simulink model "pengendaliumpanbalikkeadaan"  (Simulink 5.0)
settings: Solver=ode45  StartTime=0.0  StopTime=8.0  RelTol=1e-3

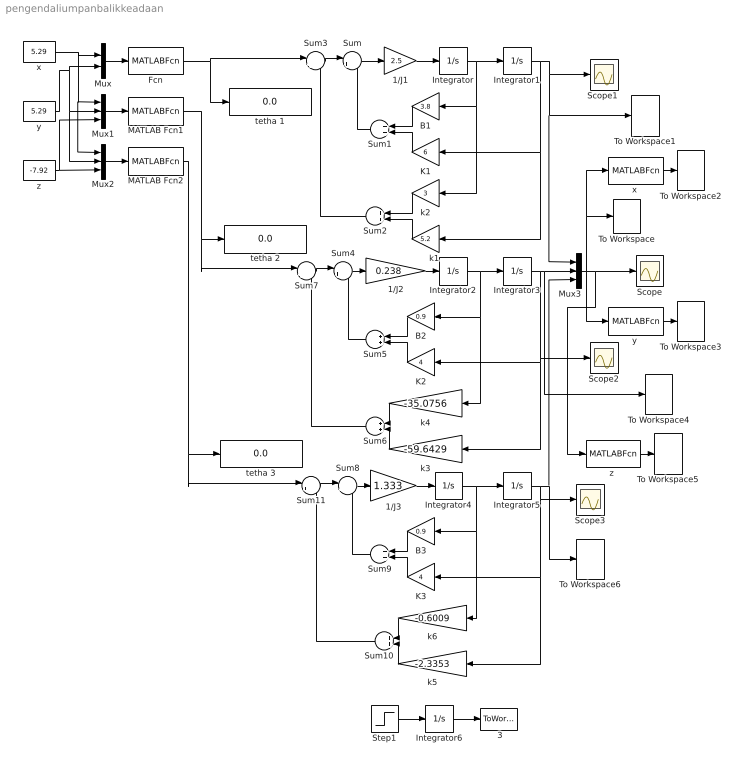
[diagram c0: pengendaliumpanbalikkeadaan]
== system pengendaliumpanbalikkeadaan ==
  " 3" : ToWorkspace  VariableName=time  SampleTime=-1  SaveFormat=Array
  1/J1 : Gain  Gain=2.5
  1/J2 : Gain  Gain=0.238
  1/J3 : Gain  Gain=1.333
  B1 : Gain  Orientation=left  Gain=3.8
  B2 : Gain  Orientation=left  Gain=0.9
  B3 : Gain  Orientation=left  Gain=0.9
  Fcn : MATLABFcn  MATLABFcn=Fcn
  Integrator{,1..6} (7 alike) : Integrator
  K1 : Gain  Orientation=left  Gain=6
  K2 : Gain  Orientation=left  Gain=4
  K3 : Gain  Orientation=left  Gain=4
  MATLAB Fcn1 : MATLABFcn  MATLABFcn=Fcn1
  MATLAB Fcn2 : MATLABFcn  MATLABFcn=Fcn2
  Mux : Mux  Inputs=2
  Mux1 : Mux  Inputs=3
  Mux2 : Mux  Inputs=3
  Mux3 : Mux  Inputs=3
  Scope : Scope
  "Scope1 " : Scope
  Scope2 : Scope
  Scope3 : Scope
  Step1 : Step  Time=0  SampleTime=0
  Sum : Sum  Inputs=|+-
  Sum{1..2,5..6,9..10} (6 alike) : Sum  Orientation=left
  Sum11 : Sum  Inputs=|++
  Sum3 : Sum  Inputs=|++
  Sum4 : Sum  Inputs=|+-
  Sum7 : Sum  Inputs=|++
  Sum8 : Sum  Inputs=|+-
  To Workspace : ToWorkspace  VariableName=yout  SampleTime=-1  SaveFormat=Array
  To Workspace1 : ToWorkspace  VariableName=u1  SampleTime=-1  SaveFormat=Array
  To Workspace2 : ToWorkspace  VariableName=xu  SampleTime=-1  SaveFormat=Array
  To Workspace3 : ToWorkspace  VariableName=yu  SampleTime=-1  SaveFormat=Array
  To Workspace4 : ToWorkspace  VariableName=u2  SampleTime=-1  SaveFormat=Array
  To Workspace5 : ToWorkspace  VariableName=zu  SampleTime=-1  SaveFormat=Array
  To Workspace6 : ToWorkspace  VariableName=u3  SampleTime=-1  SaveFormat=Array
  k1 : Gain  Orientation=left  Gain=5.2
  k2 : Gain  Orientation=left  Gain=3
  k3 : Gain  Orientation=left  Gain=-59.6429
  k4 : Gain  Orientation=left  Gain=-35.0756
  k5 : Gain  Orientation=left  Gain=-2.3353
  k6 : Gain  Orientation=left  Gain=-0.6009
  tetha 1 : Display
  tetha 2 : Display
  tetha 3 : Display
  x : Constant  Value=5.29
  "x " : MATLABFcn  MATLABFcn=x
  y : Constant  Value=5.29
  "y " : MATLABFcn  MATLABFcn=y
  z : Constant  Value=-7.92
  "z " : MATLABFcn  MATLABFcn=z
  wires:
  x/1 -> Mux1/1, Mux2/1, Mux/1
  Mux/1 -> Fcn/1
  Fcn/1 -> tetha 1/1, Sum3/1
  y/1 -> Mux2/2, Mux1/2, Mux/2
  Mux1/1 -> MATLAB Fcn1/1
  MATLAB Fcn1/1 -> tetha 2/1, Sum7/1
  MATLAB Fcn2/1 -> tetha 3/1, Sum11/1
  Mux2/1 -> MATLAB Fcn2/1
  z/1 -> Mux1/3, Mux2/3
  Sum/1 -> 1/J1/1
  1/J1/1 -> Integrator/1
  Integrator1/1 -> k1/1, K1/1, "Scope1 "/1, Mux3/1, To Workspace1/1
  Sum1/1 -> Sum/2
  B1/1 -> Sum1/1
  K1/1 -> Sum1/2
  k2/1 -> Sum2/1
  k1/1 -> Sum2/2
  Sum3/1 -> Sum/1
  Sum2/1 -> Sum3/2
  Integrator/1 -> k2/1, B1/1, Integrator1/1
  Sum4/1 -> 1/J2/1
  1/J2/1 -> Integrator2/1
  Integrator3/1 -> K2/1, k3/1, Scope2/1, Mux3/2, To Workspace4/1
  Sum5/1 -> Sum4/2
  B2/1 -> Sum5/1
  K2/1 -> Sum5/2
  k4/1 -> Sum6/1
  k3/1 -> Sum6/2
  Sum7/1 -> Sum4/1
  Sum6/1 -> Sum7/2
  Integrator2/1 -> k4/1, B2/1, Integrator3/1
  Sum8/1 -> 1/J3/1
  1/J3/1 -> Integrator4/1
  Integrator5/1 -> Scope3/1, k5/1, K3/1, Mux3/3, To Workspace6/1
  Sum9/1 -> Sum8/2
  B3/1 -> Sum9/1
  K3/1 -> Sum9/2
  k6/1 -> Sum10/1
  k5/1 -> Sum10/2
  Sum11/1 -> Sum8/1
  Sum10/1 -> Sum11/2
  Integrator4/1 -> k6/1, B3/1, Integrator5/1
  Mux3/1 -> To Workspace/1, "x "/1, "y "/1, Scope/1, "z "/1
  Step1/1 -> Integrator6/1
  Integrator6/1 -> " 3"/1
  "x "/1 -> To Workspace2/1
  "y "/1 -> To Workspace3/1
  "z "/1 -> To Workspace5/1
